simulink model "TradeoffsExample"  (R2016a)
settings: Solver=VariableStepAuto  StartTime=0.0  StopTime=Tf  RelTol=1e-7  AbsTol=1e-6
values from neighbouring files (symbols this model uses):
  Gden = [1 0]    [Section6p3_TradeoffsExample.m]    (also in Section6p5_LSComponentsExample.m = [1 2])
  Gnum = 1    [Section6p3_TradeoffsExample.m]    (also in Section6p5_LSComponentsExample.m = 5)
  Kp = 10    [Section6p3_TradeoffsExample.m]    (also in Section6p4_LoopshapingComponents.m; Section6p5_LSComponentsExample.m = 3)

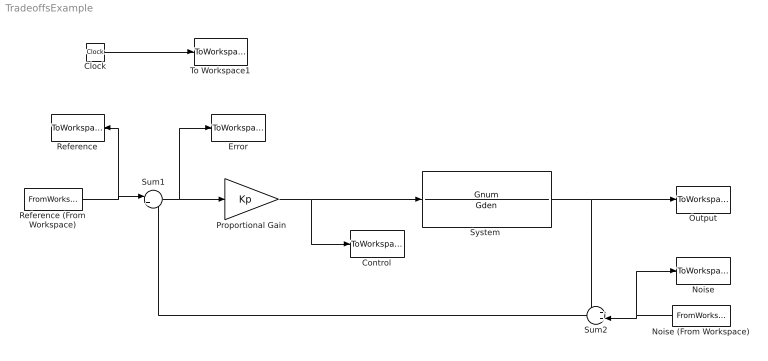
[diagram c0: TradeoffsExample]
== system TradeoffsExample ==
  Clock : Clock
  Control : ToWorkspace  VariableName=u  SampleTime=-1
  Error : ToWorkspace  VariableName=e  SampleTime=-1
  Noise : ToWorkspace  VariableName=n  SampleTime=-1
  Noise (From Workspace) : FromWorkspace  VariableName=nData  SampleTime=0
  Output : ToWorkspace  VariableName=y  SampleTime=-1
  Proportional Gain : Gain  Gain=Kp
  Reference : ToWorkspace  VariableName=r  SampleTime=-1
  Reference (From Workspace) : FromWorkspace  VariableName=rData  SampleTime=0
  Sum1 : Sum  Inputs=|+-
  Sum2 : Sum  Inputs=++|
  "System " : TransferFcn  Numerator=Gnum  Denominator=Gden
  To Workspace1 : ToWorkspace  VariableName=t  SampleTime=-1
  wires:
  Clock/1 -> To Workspace1/1
  Proportional Gain/1 -> "System "/1, Control/1
  "System "/1 -> Sum2/1, Output/1
  Sum1/1 -> Proportional Gain/1, Error/1
  Sum2/1 -> Sum1/2
  Reference (From Workspace)/1 -> Reference/1, Sum1/1
  Noise (From Workspace)/1 -> Noise/1, Sum2/2
